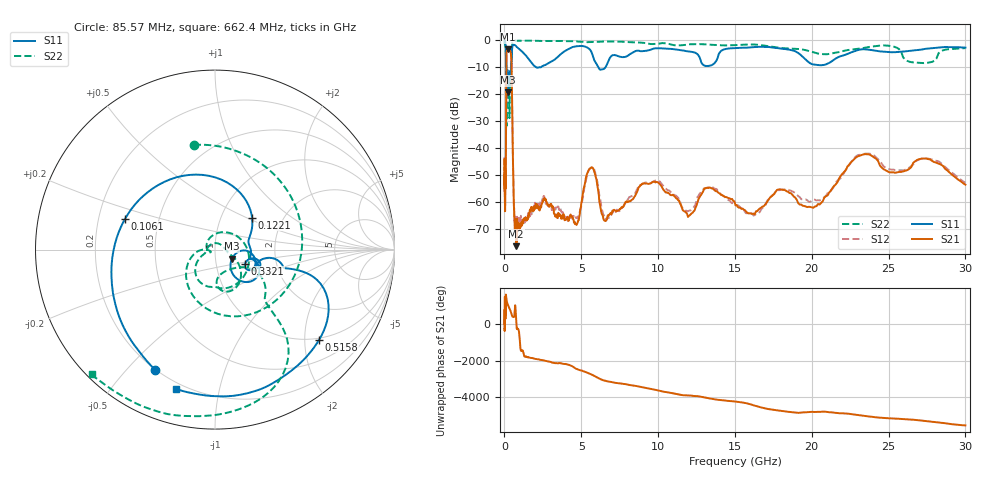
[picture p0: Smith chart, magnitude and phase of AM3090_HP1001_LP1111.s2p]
! Date/Time: Thu, Feb 28, 2019 2:03 PM
! Network Analyzer: Agilent Technologies E8364B Rev: A.07.50.67
! Sweep from 0.010 to 30.000 GHz, 1601 Points, Sweep Type: LOG
! Power Supply: 5.023 V, 0.002 A
# Hz S DB R 50
!freq MagS11 AngS11 MagS21 AngS21 MagS12 AngS12 MagS22 AngS22
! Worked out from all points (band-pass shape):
!   1601 points, 10 MHz to 30 GHz, reference 50 ohm
!   highest |S21| = -3.48 dB at 250.9 MHz (marker M1); lowest = -76.3 dB at 762.1 MHz (marker M2)
!   |S21| within 3 dB of the highest: 126.5 MHz to 442.3 MHz (315.8 MHz wide, 111 % of centre)
!   lowest |S11| = -19.4 dB at 243.5 MHz (marker M3), VSWR 1.24, Z = 60.1 - j6.08 ohm
!   |S11| at or under -10 dB: 119.9 MHz to 427.7 MHz (307.8 MHz wide, 112 % of centre); 2.033 GHz to 2.391 GHz (357.4 MHz wide, 16.2 % of centre); 6.098 GHz to 6.59 GHz (491.8 MHz wide, 7.75 % of centre)
!   |S22| runs from -31.8 to -0.2 dB; largest |S21 - S12| = 0.011
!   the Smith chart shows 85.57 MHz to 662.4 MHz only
!   S11 on the Smith chart (normalised r, x): 85.57 MHz: 0.20, -0.60; 106.1 MHz: 0.32, +0.15; 122.1 MHz: 1.40, +0.54; 332.1 MHz: 1.38, -0.23; 515.8 MHz: 0.96, -2.35; 662.4 MHz: 0.17, -0.75
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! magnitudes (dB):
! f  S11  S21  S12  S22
! 10 MHz  -0.2  -55.3  -43.9  -0.7
! 38.04 MHz  -0.5  -60.5  -60.6  -1.7
! 85.57 MHz  -2.5  -54.6  -53.0  -4.5
! 106.1 MHz  -5.5  -26.1  -26.3  -6.6
! 122.1 MHz  -11.3  -8.3  -8.2  -15.5
! 144.7 MHz  -13.9  -4.4  -4.4  -26.7
! 243.5 MHz  -19.4  -3.5  -3.4  -13.6
! 250.9 MHz  -18.7  -3.5  -3.4  -13.6
! 332.1 MHz  -14.6  -3.6  -3.6  -27.1
! 450.6 MHz  -8.0  -7.2  -7.2  -8.1
! 515.8 MHz  -2.3  -30.9  -30.7  -1.0
! 550.5 MHz  -1.9  -43.9  -43.5  -0.5
! 662.4 MHz  -1.9  -67.7  -66.6  -0.2
! 762.1 MHz  -2.4  -76.3  -66.6  -0.3
! 2.084 GHz  -10.2  -60.6  -62.1  -0.3
! 4.663 GHz  -2.3  -68.2  -65.8  -0.5
! 5.64 GHz  -4.2  -47.3  -47.2  -0.8
! 6.521 GHz  -10.5  -66.8  -65.8  -0.6
! 7.926 GHz  -6.2  -59.8  -59.9  -0.8
! 19.9 GHz  -8.6  -61.7  -59.9  -4.2
! 23.36 GHz  -3.4  -42.3  -42.2  -3.0
! 30 GHz  -2.8  -53.5  -52.8  -3.1
